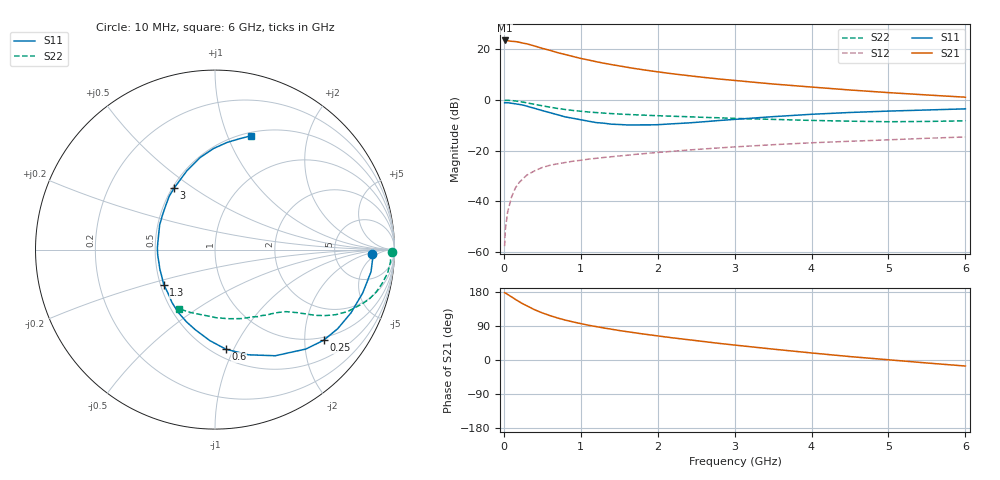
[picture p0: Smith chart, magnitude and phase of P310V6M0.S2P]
! SIEMENS Small Signal Semiconductors
! BFP181
! Si NPN RF Bipolar Junction Transistor in SOT143
! VCE = 10 V  IC = 6 mA
! Common Emitter S-Parameters:  March  1996
# GHz  S  MA  R  50
!  f  S11  S21  S12  S22
! GHz  MAG  ANG  MAG  ANG  MAG  ANG  MAG  ANG
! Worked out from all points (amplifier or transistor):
!   36 points, 10 MHz to 6 GHz, reference 50 ohm
!   highest |S21| = 23.4 dB at 10 MHz (marker M1)
!   |S21| within 3 dB of that: start of sweep to 487.1 MHz
!   unconditionally stable (mu >= 1): 1.757 GHz to end of sweep
!   at 250 MHz: K = 0.23, MSG = 26.7 dB, |S12| = -31.1 dB
!   at 1.4 GHz: K = 0.90, MSG = 18.2 dB, |S12| = -22.4 dB
!   at 6 GHz: K = 1.06, MAG = 6.3 dB, |S12| = -14.6 dB
!   S11 on the Smith chart (normalised r, x): 10 MHz: 15, -3; 250 MHz: 0.92, -2.45; 600 MHz: 0.58, -0.93; 1.3 GHz: 0.52, -0.23; 3 GHz: 0.51, +0.42; 6 GHz: 0.54, +1.22
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0.01  0.877 -1.7  14.86 177.6  0.0013 66.3  0.9853 -0.7
0.02  0.8797 -3.5  14.85 176.9  0.0028 85.8  0.9772 -1.4
0.05  0.8781 -8.1  14.7 172.9  0.0062 86.5  0.9804 -3.9
0.15  0.8355 -25.0  14.15 160.0  0.0183 75.4  0.9511 -11.3
0.2  0.8131 -32.9  13.72 153.9  0.0235 71.4  0.929 -14.7
0.25  0.7881 -39.9  13.14 147.9  0.028 68.7  0.903 -17.7
0.3  0.7504 -47.6  12.75 142.9  0.0329 65.0  0.8733 -20.3
0.4  0.6801 -60.4  11.55 132.6  0.0398 59.7  0.816 -25.0
0.5  0.6149 -72.4  10.38 124.3  0.0464 55.1  0.7646 -28.3
0.6  0.5585 -83.7  9.482 117.1  0.0512 51.8  0.7178 -30.8
0.7  0.5081 -93.2  8.531 110.8  0.0549 49.6  0.677 -32.8
0.8  0.4606 -103.6  7.833 105.2  0.0582 47.2  0.6451 -34.2
0.9  0.4329 -111.5  7.169 100.5  0.0617 46.0  0.6178 -35.4
1.1  0.3797 -129.2  6.119 91.7  0.0677 43.9  0.5769 -37.5
1.3  0.3464 -145.5  5.284 84.5  0.0731 42.6  0.5485 -39.3
1.7  0.3206 -174.7  4.157 71.9  0.0838 41.0  0.5081 -43.3
2.2  0.3377 155.9  3.262 58.3  0.0969 38.8  0.4746 -49.0
3  0.4119 123.5  2.416 39.4  0.118 34.2  0.4311 -60.3
3.5  0.4664 109.6  2.056 28.7  0.1305 31.0  0.4121 -68.9
4.5  0.5639 90.7  1.566 9.0  0.1526 23.6  0.3798 -88.9
5.5  0.6316 77.7  1.25 -7.9  0.1746 17.5  0.3753 -110.2
6  0.6648 72.5  1.129 -15.9  0.1855 13.8  0.3861 -121.3
